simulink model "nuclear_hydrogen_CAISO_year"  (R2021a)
settings: Solver=ode23s  StartTime=0  StopTime=31618800  MaxStep=60  RelTol=2e-3
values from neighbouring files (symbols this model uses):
  alpha_f = -1.98e-5/beta    (= -0.00282857142857)    [parameter_s5.m]
  alpha_m = -28.2e-5/beta    (= -0.0402857142857)    [parameter_s5.m]
  As = n_rod*(height*2*pi*r_pellet + 2*pi*r_pellet^2)    (= 584.56254954)    [parameter_s5.m]
  beta = 0.0070    (= 0.007)    [parameter_s5.m]    (also in XSteam.m = 0)
  Cp_H2 = readmatrix('Cp.xlsx')    [parameter_s5.m]
  Ef = 200.7*1.6022e-13    (= 3.2156154e-11)    [parameter_s5.m]
  h = Nu*kappa_m/Dh    (= 9811.48906394)    [parameter_s5.m]    (also in XSteam.m = [5219.76331549428,5206.09634477373,6583.80290533381])
  k_H2 = xlsread('Hydrogen thermal conductivities.xlsx')    [parameter_s5.m]
  Lambda = 2.18e-5    (= 2.18e-05)    [parameter_s5.m]
  lambdaC = 7.728e-2    (= 0.07728)    [parameter_s5.m]
  m = Mf*1000*4/100    (= 368875.1038)    [parameter_s5.m]
  Mf = 37*249.239935    (= 9221.877595)    [parameter_s5.m]
  Mm = rho_m*V    (= 10677.6636904)    [parameter_s5.m]
  mu_H2 = xlsread('Hydrogen density.xlsx')    [parameter_s5.m]
  MW = 235.043    [parameter_s5.m]
  NA = 6.0221409e23    (= 6.0221409e+23)    [parameter_s5.m]
  p0 = -0.0065    [parameter_s5.m]
  p1 = -0.440    (= -0.44)    [parameter_s5.m]    (also in XSteam.m = p1_hs(h, s))
  p2 = -0.966    [parameter_s5.m]    (also in XSteam.m = p2_hs(h, s))
  phi0 = 9.04e+12    (= 9040000000000)    [parameter_s5.m]
  r_clad = 0.0609e-2    (= 0.000609)    [parameter_s5.m]
  r_pellet = 0.4751e-2    (= 0.004751)    [parameter_s5.m]
  rho_H2 = xlsread('Hydrogen density.xlsx')    [parameter_s5.m]
  sigmaN = 585e-24    (= 5.85e-22)    [parameter_s5.m]
  Tf0 = 719    [parameter_s5.m]
  Tm0 = 283.37    [parameter_s5.m]
libraries: pid_lib x4

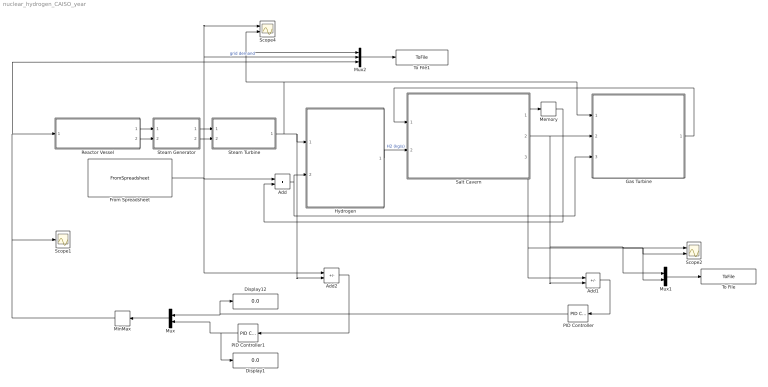
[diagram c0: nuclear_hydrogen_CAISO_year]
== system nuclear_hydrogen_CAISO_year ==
  Add : Sum
  Add1 : Sum  Inputs=+-
  Add2 : Sum  Inputs=+-
  Display1 : Display
  Display12 : Display
  From Spreadsheet : FromSpreadsheet  FileName=HistoricalEMSHourlyLoad-2020.xlsx  SheetName=data
  Gas Turbine : Subsystem
  Hydrogen : Subsystem
  Memory : Memory
  MinMax : MinMax
  Mux : Mux  Inputs=2
  Mux1 : Mux  Inputs=2
  Mux2 : Mux  Inputs=3
  PID Controller : pid_lib/PID Controller  Controller=PID  Form=Parallel  TimeDomain=Continuous-time  UseExternalTs=off  SampleTime=-1  IntegratorMethod=Forward Euler  FilterMethod=Forward Euler  ControllerParametersSource=internal  P=-1e-7  I=-5e-8  D=0  UseFilter=on  N=100  TunerSelectOption=Transfer Function Based (PID Tuner App)  InitialConditionSource=internal  InitialConditionForIntegrator=0  InitialConditionForFilter=0  DifferentiatorICPrevScaledInput=0  ExternalReset=none  TrackingMode=off  Kt=1  LimitOutput=on  SatLimitsSource=internal  UpperSaturationLimit=2  LowerSaturationLimit=0  LinearizeAsGain=on  AntiWindupMode=clamping  Kb=1  POutMin=[]  POutMax=[]  IOutMin=[]  IOutMax=[]  DOutMin=[]  DOutMax=[]  NOutMin=[]  NOutMax=[]  SumOutMin=[]  SumOutMax=[]  SaturationOutMin=[]  SaturationOutMax=[]  PParamMin=[]  PParamMax=[]  IParamMin=[]  IParamMax=[]  DParamMin=[]  DParamMax=[]  NParamMin=[]  NParamMax=[]  KbParamMin=[]  KbParamMax=[]  KtParamMin=[]  KtParamMax=[]  KbOutMin=[]  KbOutMax=[]  KtOutMin=[]  KtOutMax=[]  IntegratorOutMin=[]  IntegratorOutMax=[]  FilterOutMin=[]  FilterOutMax=[]  SumI1OutMin=[]  SumI1OutMax=[]  SumI2OutMin=[]  SumI2OutMax=[]  SumI3OutMin=[]  SumI3OutMax=[]  SumI4OutMin=[]  SumI4OutMax=[]  SumDOutMin=[]  SumDOutMax=[]  DifferentiatorOutMin=[]  DifferentiatorOutMax=[]  FilterDiffOutCoefMin=[]  FilterDiffOutCoefMax=[]  ReciprocalOutMin=[]  ReciprocalOutMax=[]  SumDenOutMin=[]  SumDenOutMax=[]  SumNumOutMin=[]  SumNumOutMax=[]  DivideOutMin=[]  DivideOutMax=[]  UdiffTsProdOutMin=[]  UdiffTsProdOutMax=[]  NTsProdOutMin=[]  NTsProdOutMax=[]  UintegralTsProdOutMin=[]  UintegralTsProdOutMax=[]  UngainTsProdOutMin=[]  UngainTsProdOutMax=[]  IntegratorContinuousStateAttributes=''  IntegratorStateMustResolveToSignalObject=off  IntegratorRTWStateStorageClass=Auto  FilterContinuousStateAttributes=''  FilterStateMustResolveToSignalObject=off  FilterRTWStateStorageClass=Auto  ParallelPVariant=InternalParameters  IdealPVariant=Disabled  IVariant=InternalParameters  DVariant=InternalParameters  IntegratorVariant=Continuous  SatVariant=Enabled  AWVariant=ContClampingParallel  PCopyVariant=Disabled  TRVariant=Disabled  FdbkBlocksVariant=Forward  IdealPFdbkVariant=Disabled  SatFdbkVariant=Disabled  DerivativeFilterVariant=ContFilter  NVariant=InternalParameters  NCopyVariant=Disabled  FilterICVariant=InternalICsFilter  IntegratorICVariant=InternalICs  ExternalResetVariant=Disabled  TRSumVariant=Passthrough  SumFdbkVariant=Disabled  SumVariant=Sum_PID  TsampFilterVariant=InternalTs  TsampNgainVariant=Passthrough  TsampIntegralVariant=Passthrough  ExternalSaturationOutDataTypeStr=Inherit: Same as second input
  PID Controller1 : pid_lib/PID Controller  Controller=PID  Form=Parallel  TimeDomain=Continuous-time  UseExternalTs=off  SampleTime=-1  IntegratorMethod=Forward Euler  FilterMethod=Forward Euler  ControllerParametersSource=internal  P=-0.067  I=-0.0044  D=0  UseFilter=on  N=100  TunerSelectOption=Transfer Function Based (PID Tuner App)  InitialConditionSource=internal  InitialConditionForIntegrator=0  InitialConditionForFilter=0  DifferentiatorICPrevScaledInput=0  ExternalReset=none  TrackingMode=off  Kt=1  LimitOutput=on  SatLimitsSource=internal  UpperSaturationLimit=2  LowerSaturationLimit=0  LinearizeAsGain=on  AntiWindupMode=clamping  Kb=1  POutMin=[]  POutMax=[]  IOutMin=[]  IOutMax=[]  DOutMin=[]  DOutMax=[]  NOutMin=[]  NOutMax=[]  SumOutMin=[]  SumOutMax=[]  SaturationOutMin=[]  SaturationOutMax=[]  PParamMin=[]  PParamMax=[]  IParamMin=[]  IParamMax=[]  DParamMin=[]  DParamMax=[]  NParamMin=[]  NParamMax=[]  KbParamMin=[]  KbParamMax=[]  KtParamMin=[]  KtParamMax=[]  KbOutMin=[]  KbOutMax=[]  KtOutMin=[]  KtOutMax=[]  IntegratorOutMin=[]  IntegratorOutMax=[]  FilterOutMin=[]  FilterOutMax=[]  SumI1OutMin=[]  SumI1OutMax=[]  SumI2OutMin=[]  SumI2OutMax=[]  SumI3OutMin=[]  SumI3OutMax=[]  SumI4OutMin=[]  SumI4OutMax=[]  SumDOutMin=[]  SumDOutMax=[]  DifferentiatorOutMin=[]  DifferentiatorOutMax=[]  FilterDiffOutCoefMin=[]  FilterDiffOutCoefMax=[]  ReciprocalOutMin=[]  ReciprocalOutMax=[]  SumDenOutMin=[]  SumDenOutMax=[]  SumNumOutMin=[]  SumNumOutMax=[]  DivideOutMin=[]  DivideOutMax=[]  UdiffTsProdOutMin=[]  UdiffTsProdOutMax=[]  NTsProdOutMin=[]  NTsProdOutMax=[]  UintegralTsProdOutMin=[]  UintegralTsProdOutMax=[]  UngainTsProdOutMin=[]  UngainTsProdOutMax=[]  IntegratorContinuousStateAttributes=''  IntegratorStateMustResolveToSignalObject=off  IntegratorRTWStateStorageClass=Auto  FilterContinuousStateAttributes=''  FilterStateMustResolveToSignalObject=off  FilterRTWStateStorageClass=Auto  ParallelPVariant=InternalParameters  IdealPVariant=Disabled  IVariant=InternalParameters  DVariant=InternalParameters  IntegratorVariant=Continuous  SatVariant=Enabled  AWVariant=ContClampingParallel  PCopyVariant=Disabled  TRVariant=Disabled  FdbkBlocksVariant=Forward  IdealPFdbkVariant=Disabled  SatFdbkVariant=Disabled  DerivativeFilterVariant=ContFilter  NVariant=InternalParameters  NCopyVariant=Disabled  FilterICVariant=InternalICsFilter  IntegratorICVariant=InternalICs  ExternalResetVariant=Disabled  TRSumVariant=Passthrough  SumFdbkVariant=Disabled  SumVariant=Sum_PID  TsampFilterVariant=InternalTs  TsampNgainVariant=Passthrough  TsampIntegralVariant=Passthrough  ExternalSaturationOutDataTypeStr=Inherit: Same as second input
  Reactor Vessel : Subsystem
  Salt Cavern : Subsystem
  Scope1 : Scope
  Scope2 : Scope  NumInputPorts=2
  Scope4 : Scope  NumInputPorts=2
  Steam Generator : Subsystem
  Steam Turbine : Subsystem
  To File : ToFile  Filename=CAISO_Cavern_Pressure_year.mat  MatrixName=ans_Pcav  SaveFormat=Timeseries
  To File1 : ToFile  Filename=CAISO_nuclear_year.mat  MatrixName=ans_NR  SaveFormat=Timeseries
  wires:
  Reactor Vessel/2(Tm) -> Steam Generator/2(Tmin)
  Reactor Vessel/1(mdot_l) -> Steam Generator/1(mdot_l)
  Hydrogen/1(Total_H2) -> Salt Cavern/2(H2_in (kg/s))  "H2 (kg/s)"
  MinMax/1 -> Scope1/1, Mux2/3, Reactor Vessel/1(control rod position (m))
  Steam Generator/1(T_steam) -> Steam Turbine/1(T1_in)
  Steam Generator/2(m_steam) -> Steam Turbine/2(m_steam)
  Add/1 -> Gas Turbine/3(grid_demand), Hydrogen/2(demand)
  Salt Cavern/1(Power_comp) -> Memory/1
  Memory/1 -> Add/2
  From Spreadsheet/1 -> Mux2/2, Scope4/1, Add2/1, Add/1  "grid demand"
  Gas Turbine/1(m_fuel) -> Salt Cavern/1(H2_out (kg/s))
  PID Controller/1 -> Display12/1, Mux/1
  PID Controller1/1 -> Display1/1, Mux/2
  Mux/1 -> MinMax/1
  Add2/1 -> PID Controller1/1
  Add1/1 -> PID Controller/1
  Salt Cavern/2(Cavern Pressure) -> Add1/2, Mux1/1, Scope2/1, Gas Turbine/2(Cavern_Pressure)
  Mux1/1 -> To File/1
  Steam Turbine/1(W_Rankine) -> Hydrogen/1(W_Rankine), Add2/2, Gas Turbine/1(Steam_Turb), Scope4/2, Mux2/1
  Mux2/1 -> To File1/1
  Salt Cavern/3(Max Pressure) -> Mux1/2, Scope2/2, Add1/1

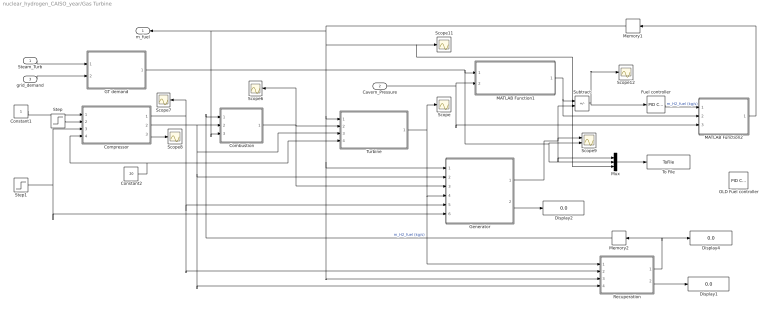
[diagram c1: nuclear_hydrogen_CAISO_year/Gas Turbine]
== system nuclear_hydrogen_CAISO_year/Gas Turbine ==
  Steam_Turb : Inport
  Cavern_Pressure : Inport  Port=2
  grid_demand : Inport  Port=3
  Combustion : MATLAB Function  TreatAsAtomicUnit=on
  Compressor : MATLAB Function  TreatAsAtomicUnit=on
  Constant1 : Constant
  Constant2 : Constant  Value=20
  Display1 : Display
  Display2 : Display
  Display4 : Display
  Fuel controller : pid_lib/PID Controller  Controller=PID  Form=Ideal  TimeDomain=Continuous-time  UseExternalTs=off  SampleTime=-1  IntegratorMethod=Forward Euler  FilterMethod=Forward Euler  ControllerParametersSource=internal  P=1e-4  I=1.2e-1  D=0  UseFilter=on  N=100  TunerSelectOption=Frequency Response Based  InitialConditionSource=internal  InitialConditionForIntegrator=0  InitialConditionForFilter=0  DifferentiatorICPrevScaledInput=0  ExternalReset=none  TrackingMode=off  Kt=1  LimitOutput=on  SatLimitsSource=internal  UpperSaturationLimit=0.2  LowerSaturationLimit=0.05236  LinearizeAsGain=on  AntiWindupMode=clamping  Kb=1  POutMin=[]  POutMax=[]  IOutMin=[]  IOutMax=[]  DOutMin=[]  DOutMax=[]  NOutMin=[]  NOutMax=[]  SumOutMin=[]  SumOutMax=[]  SaturationOutMin=[]  SaturationOutMax=[]  PParamMin=[]  PParamMax=[]  IParamMin=[]  IParamMax=[]  DParamMin=[]  DParamMax=[]  NParamMin=[]  NParamMax=[]  KbParamMin=[]  KbParamMax=[]  KtParamMin=[]  KtParamMax=[]  KbOutMin=[]  KbOutMax=[]  KtOutMin=[]  KtOutMax=[]  IntegratorOutMin=[]  IntegratorOutMax=[]  FilterOutMin=[]  FilterOutMax=[]  SumI1OutMin=[]  SumI1OutMax=[]  SumI2OutMin=[]  SumI2OutMax=[]  SumI3OutMin=[]  SumI3OutMax=[]  SumI4OutMin=[]  SumI4OutMax=[]  SumDOutMin=[]  SumDOutMax=[]  DifferentiatorOutMin=[]  DifferentiatorOutMax=[]  FilterDiffOutCoefMin=[]  FilterDiffOutCoefMax=[]  ReciprocalOutMin=[]  ReciprocalOutMax=[]  SumDenOutMin=[]  SumDenOutMax=[]  SumNumOutMin=[]  SumNumOutMax=[]  DivideOutMin=[]  DivideOutMax=[]  UdiffTsProdOutMin=[]  UdiffTsProdOutMax=[]  NTsProdOutMin=[]  NTsProdOutMax=[]  UintegralTsProdOutMin=[]  UintegralTsProdOutMax=[]  UngainTsProdOutMin=[]  UngainTsProdOutMax=[]  IntegratorContinuousStateAttributes=''  IntegratorStateMustResolveToSignalObject=off  IntegratorRTWStateStorageClass=Auto  FilterContinuousStateAttributes=''  FilterStateMustResolveToSignalObject=off  FilterRTWStateStorageClass=Auto  ParallelPVariant=Passthrough  IdealPVariant=InternalParameters  IVariant=InternalParameters  DVariant=InternalParameters  IntegratorVariant=Continuous  SatVariant=Enabled  AWVariant=ContClampingIdeal  PCopyVariant=InternalParamsIdeal  TRVariant=Disabled  FdbkBlocksVariant=Forward  IdealPFdbkVariant=Disabled  SatFdbkVariant=Disabled  DerivativeFilterVariant=ContFilter  NVariant=InternalParameters  NCopyVariant=Disabled  FilterICVariant=InternalICsFilter  IntegratorICVariant=InternalICs  ExternalResetVariant=Disabled  TRSumVariant=Passthrough  SumFdbkVariant=Disabled  SumVariant=Sum_PID  TsampFilterVariant=InternalTs  TsampNgainVariant=Passthrough  TsampIntegralVariant=Passthrough  ExternalSaturationOutDataTypeStr=Inherit: Same as second input
  GT demand : MATLAB Function  TreatAsAtomicUnit=on
  Generator : MATLAB Function  TreatAsAtomicUnit=on
  MATLAB Function1 : MATLAB Function  TreatAsAtomicUnit=on
  MATLAB Function2 : MATLAB Function  TreatAsAtomicUnit=on
  Memory1 : Memory
  Memory2 : Memory
  Mux : Mux  Inputs=3
  OLD Fuel controller : pid_lib/PID Controller  Controller=PID  Form=Ideal  TimeDomain=Continuous-time  UseExternalTs=off  SampleTime=-1  IntegratorMethod=Forward Euler  FilterMethod=Forward Euler  ControllerParametersSource=internal  P=1e-3  I=1e-2  D=0  UseFilter=on  N=100  TunerSelectOption=Frequency Response Based  InitialConditionSource=internal  InitialConditionForIntegrator=0  InitialConditionForFilter=0  DifferentiatorICPrevScaledInput=0  ExternalReset=none  TrackingMode=off  Kt=1  LimitOutput=on  SatLimitsSource=internal  UpperSaturationLimit=0.2  LowerSaturationLimit=0.05236  LinearizeAsGain=on  AntiWindupMode=clamping  Kb=1  POutMin=[]  POutMax=[]  IOutMin=[]  IOutMax=[]  DOutMin=[]  DOutMax=[]  NOutMin=[]  NOutMax=[]  SumOutMin=[]  SumOutMax=[]  SaturationOutMin=[]  SaturationOutMax=[]  PParamMin=[]  PParamMax=[]  IParamMin=[]  IParamMax=[]  DParamMin=[]  DParamMax=[]  NParamMin=[]  NParamMax=[]  KbParamMin=[]  KbParamMax=[]  KtParamMin=[]  KtParamMax=[]  KbOutMin=[]  KbOutMax=[]  KtOutMin=[]  KtOutMax=[]  IntegratorOutMin=[]  IntegratorOutMax=[]  FilterOutMin=[]  FilterOutMax=[]  SumI1OutMin=[]  SumI1OutMax=[]  SumI2OutMin=[]  SumI2OutMax=[]  SumI3OutMin=[]  SumI3OutMax=[]  SumI4OutMin=[]  SumI4OutMax=[]  SumDOutMin=[]  SumDOutMax=[]  DifferentiatorOutMin=[]  DifferentiatorOutMax=[]  FilterDiffOutCoefMin=[]  FilterDiffOutCoefMax=[]  ReciprocalOutMin=[]  ReciprocalOutMax=[]  SumDenOutMin=[]  SumDenOutMax=[]  SumNumOutMin=[]  SumNumOutMax=[]  DivideOutMin=[]  DivideOutMax=[]  UdiffTsProdOutMin=[]  UdiffTsProdOutMax=[]  NTsProdOutMin=[]  NTsProdOutMax=[]  UintegralTsProdOutMin=[]  UintegralTsProdOutMax=[]  UngainTsProdOutMin=[]  UngainTsProdOutMax=[]  IntegratorContinuousStateAttributes=''  IntegratorStateMustResolveToSignalObject=off  IntegratorRTWStateStorageClass=Auto  FilterContinuousStateAttributes=''  FilterStateMustResolveToSignalObject=off  FilterRTWStateStorageClass=Auto  ParallelPVariant=Passthrough  IdealPVariant=InternalParameters  IVariant=InternalParameters  DVariant=InternalParameters  IntegratorVariant=Continuous  SatVariant=Enabled  AWVariant=ContClampingIdeal  PCopyVariant=InternalParamsIdeal  TRVariant=Disabled  FdbkBlocksVariant=Forward  IdealPFdbkVariant=Disabled  SatFdbkVariant=Disabled  DerivativeFilterVariant=ContFilter  NVariant=InternalParameters  NCopyVariant=Disabled  FilterICVariant=InternalICsFilter  IntegratorICVariant=InternalICs  ExternalResetVariant=Disabled  TRSumVariant=Passthrough  SumFdbkVariant=Disabled  SumVariant=Sum_PID  TsampFilterVariant=InternalTs  TsampNgainVariant=Passthrough  TsampIntegralVariant=Passthrough  ExternalSaturationOutDataTypeStr=Inherit: Same as second input
  Recuperation : MATLAB Function  TreatAsAtomicUnit=on
  Scope{,6..8,11..12} (6 alike) : Scope
  Scope9 : Scope  NumInputPorts=2
  Step : Step  Time=4  Before=80  After=80  SampleTime=0
  Step1 : Step  Time=7  Before=280  After=280  SampleTime=0
  Subtract : Sum  Inputs=+-
  To File : ToFile  Filename=CAISO_GT_Power_year.mat  MatrixName=ans_GT  SaveFormat=Timeseries
  Turbine : MATLAB Function  TreatAsAtomicUnit=on
  m_fuel : Outport
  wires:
  Combustion/1(T_f) -> Generator/3(T_f), Scope6/1, Turbine/2(T_f)
  Constant2/1 -> Compressor/4(m_an), Turbine/4(m_an)
  GT demand/1(GT_demand) -> Mux/2, Scope9/2, MATLAB Function1/1(SP)
  Fuel controller/1 -> MATLAB Function2/1(m_f)  "m_H2_fuel (kg/s)"
  MATLAB Function1/1(Set_point) -> MATLAB Function2/2(GT_SP), Subtract/1
  Generator/1(P_overall) -> Mux/1, Scope9/1, Subtract/2
  Steam_Turb/1 -> GT demand/1(Steam_Turb)
  Cavern_Pressure/1 -> MATLAB Function2/3(Cavern_P), MATLAB Function1/2(Cavern_Pressure)
  Step1/1 -> Generator/6(T_amb), Compressor/3(T_amb)
  Constant1/1 -> Compressor/1(P_amb)
  Subtract/1 -> Scope12/1, Fuel controller/1
  Step/1 -> Compressor/2(theta_IGV)
  Compressor/3(P_out) -> Scope8/1
  grid_demand/1 -> GT demand/2(grid_demand)
  Compressor/1(Td) -> Recuperation/2(T_d), Generator/5(T_d), Scope7/1
  Turbine/1(T_e) -> Scope/1, Recuperation/1(T_e), Generator/4(T_e)
  Recuperation/1(Tc_in) -> Display4/1, Memory2/1
  Compressor/2(m_a) -> Recuperation/4(m_a), Generator/2(m_a), Turbine/3(m_a), Combustion/2(m_a)
  Memory2/1 -> Combustion/1(T_d)  "m_H2_fuel (kg/s)"
  Recuperation/2(T_6) -> Display1/1
  Generator/2(efficiency) -> Display2/1
  Mux/1 -> To File/1
  Memory1/1 -> Combustion/3(m_f), m_fuel/1, Mux/3, Scope11/1, Recuperation/3(m_f), Generator/1(m_f), Turbine/1(m_f)
  MATLAB Function2/1(m_H2) -> Memory1/1

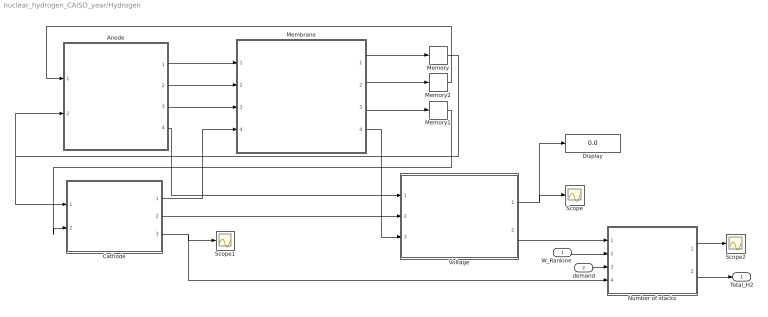
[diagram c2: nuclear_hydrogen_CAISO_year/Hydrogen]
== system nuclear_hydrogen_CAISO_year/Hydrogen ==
  W_Rankine : Inport
  demand : Inport  Port=2
  Anode : MATLAB Function  TreatAsAtomicUnit=on
  Cathode : MATLAB Function  TreatAsAtomicUnit=on
  Display : Display
  Membrane : MATLAB Function  TreatAsAtomicUnit=on
  Memory : Memory
  Memory1 : Memory
  Memory2 : Memory
  Number of stacks : MATLAB Function  TreatAsAtomicUnit=on
  Scope : Scope
  Scope1 : Scope
  Scope2 : Scope
  Voltage : MATLAB Function  TreatAsAtomicUnit=on
  Total_H2 : Outport
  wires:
  Memory/1 -> Anode/2(F_H2O_m), Cathode/1(F_H2O_m)
  Cathode/1(nH2O_cat) -> Membrane/4(n_H2O_c)
  Anode/1(nH2O_an) -> Membrane/1(n_H2O_a)
  Membrane/1(FH2Om) -> Memory/1
  Cathode/2(P_H2) -> Voltage/2(P_H2)
  Cathode/3(dNH2dt) -> Number of stacks/4(n_H2), Scope1/1
  Memory1/1 -> Cathode/2(D_cat)
  Memory2/1 -> Anode/1(D_an)
  Anode/4(P_O2) -> Voltage/1(P_O2)
  Voltage/1(V) -> Display/1, Scope/1
  Membrane/3(D_cat) -> Memory1/1
  Membrane/2(D_an) -> Memory2/1
  Membrane/4(PH2O_me_an) -> Voltage/3(P_H2O)
  Anode/2(F_H2O_cons) -> Membrane/2(FH2O_cons)
  Anode/3(CO2_me) -> Membrane/3(CO2_me)
  Voltage/2(Power) -> Number of stacks/1(Power)
  W_Rankine/1 -> Number of stacks/2(P_Turb)
  Number of stacks/2(Total_H2) -> Total_H2/1
  demand/1 -> Number of stacks/3(demand)
  Number of stacks/1(n) -> Scope2/1

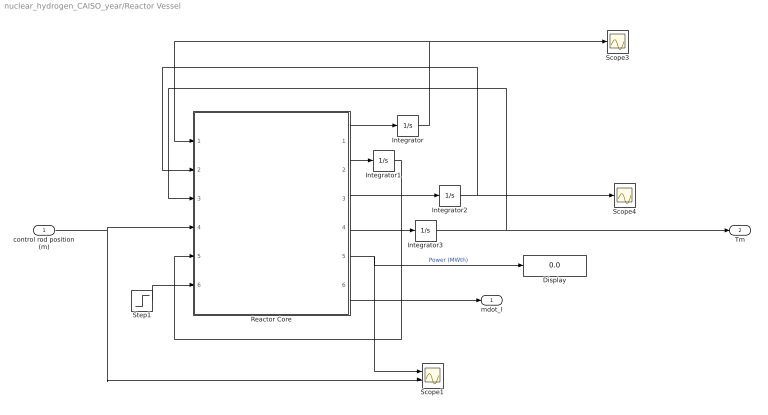
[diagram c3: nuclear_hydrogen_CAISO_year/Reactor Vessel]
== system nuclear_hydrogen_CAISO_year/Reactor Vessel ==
  control rod position (m) : Inport
  Display : Display
  Integrator : Integrator  InitialCondition=99.35
  Integrator1 : Integrator  InitialCondition=.65
  Integrator2 : Integrator  InitialCondition=719
  Integrator3 : Integrator  InitialCondition=284
  Reactor Core : MATLAB Function  TreatAsAtomicUnit=on
  Scope1 : Scope  NumInputPorts=2
  Scope3 : Scope
  Scope4 : Scope
  Step1 : Step  Time=6  Before=258.3  After=258.3  SampleTime=0
  mdot_l : Outport
  Tm : Outport  Port=2
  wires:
  Integrator1/1 -> Reactor Core/5(C)
  Integrator2/1 -> Scope4/1, Reactor Core/2(Tf)
  Integrator/1 -> Reactor Core/1(N), Scope3/1
  Reactor Core/2(dCdt) -> Integrator1/1
  Reactor Core/1(dNdt) -> Integrator/1
  Reactor Core/5(Power) -> Scope1/1, Display/1  "Power (MWth)"
  control rod position (m)/1 -> Scope1/2, Reactor Core/4(z)
  Reactor Core/3(dTfdt) -> Integrator2/1
  Integrator3/1 -> Tm/1, Reactor Core/3(Tm)
  Reactor Core/4(dTmdt) -> Integrator3/1
  Step1/1 -> Reactor Core/6(Tin)
  Reactor Core/6(mdot_l) -> mdot_l/1

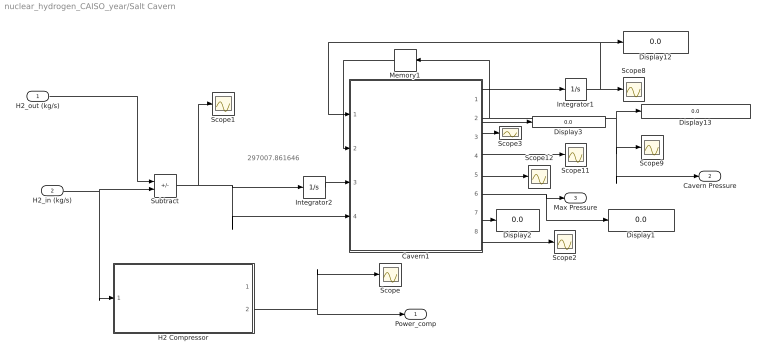
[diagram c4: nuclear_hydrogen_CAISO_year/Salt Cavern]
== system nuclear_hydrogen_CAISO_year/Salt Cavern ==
  note: 297007.861646
  H2_out (kg/s) : Inport
  H2_in (kg/s) : Inport  Port=2
  Cavern1 : MATLAB Function  TreatAsAtomicUnit=on
  Display{1..3,12..13} (5 alike) : Display
  H2 Compressor : MATLAB Function  TreatAsAtomicUnit=on
  Integrator1 : Integrator  InitialCondition=313.15
  Integrator2 : Integrator  InitialCondition=297007.861646
  Memory1 : Memory
  Scope{,1..3,8..9,11..12} (8 alike) : Scope
  Subtract : Sum  Inputs=-+
  Power_comp : Outport
  Cavern Pressure : Outport  Port=2
  Max Pressure : Outport  Port=3
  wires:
  Cavern1/4(z) -> Scope11/1
  Cavern1/2(P) -> Cavern Pressure/1, Scope9/1, Display13/1, Memory1/1
  H2_in (kg/s)/1 -> H2 Compressor/1(nH2), Subtract/2
  Cavern1/1(dTdt) -> Integrator1/1
  Integrator1/1 -> Scope8/1, Display12/1, Cavern1/1(T)
  Memory1/1 -> Cavern1/2("P ")
  Integrator2/1 -> Cavern1/3(m)
  Cavern1/5(lambda) -> Scope12/1
  H2 Compressor/2(Total_P) -> Scope/1, Power_comp/1
  H2_out (kg/s)/1 -> Subtract/1
  Subtract/1 -> Scope1/1, Integrator2/1, Cavern1/4(mH2_in)
  Cavern1/6(P_max) -> Display1/1, Max Pressure/1
  Cavern1/7(P_min) -> Display2/1
  Cavern1/8(Cp) -> Scope2/1
  Cavern1/3(n) -> Display3/1, Scope3/1

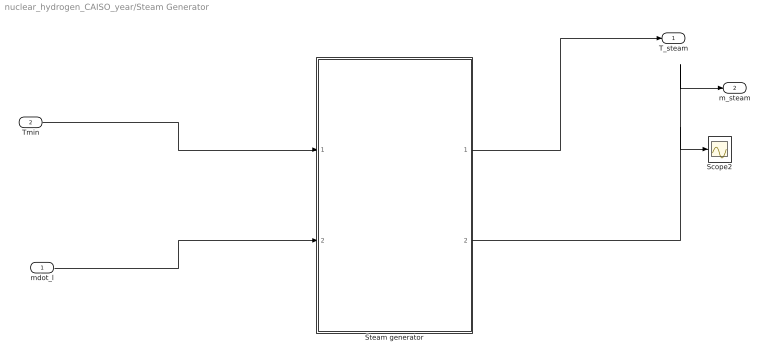
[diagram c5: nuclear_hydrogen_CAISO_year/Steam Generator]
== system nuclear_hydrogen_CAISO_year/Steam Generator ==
  mdot_l : Inport
  Tmin : Inport  Port=2
  Scope2 : Scope
  Steam generator : MATLAB Function  TreatAsAtomicUnit=on
  T_steam : Outport
  m_steam : Outport  Port=2
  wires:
  Steam generator/2(m_steam) -> m_steam/1, Scope2/1
  Tmin/1 -> Steam generator/1(Tmin)
  mdot_l/1 -> Steam generator/2(mdot_l)
  Steam generator/1(T_steam_out) -> T_steam/1

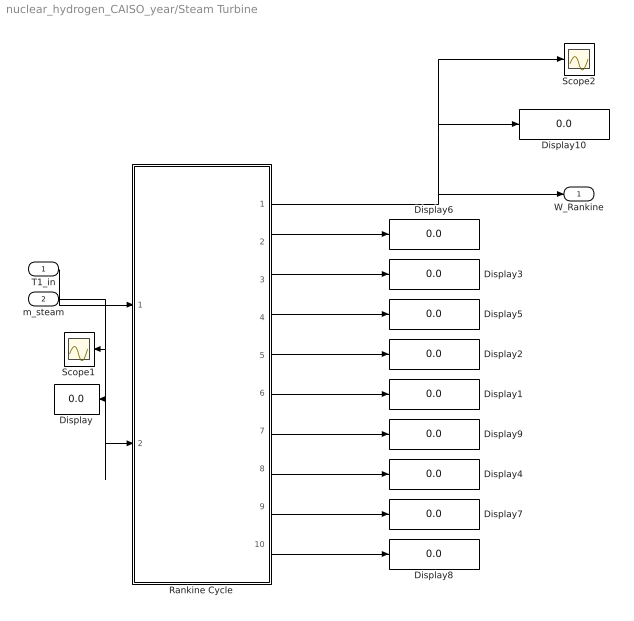
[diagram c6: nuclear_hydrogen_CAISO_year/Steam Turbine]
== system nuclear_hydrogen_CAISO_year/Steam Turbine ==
  T1_in : Inport
  m_steam : Inport  Port=2
  Display{,1..10} (11 alike) : Display
  Rankine Cycle : MATLAB Function  TreatAsAtomicUnit=on
  Scope1 : Scope
  Scope2 : Scope
  W_Rankine : Outport
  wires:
  Rankine Cycle/2(W_T1) -> Display6/1
  Rankine Cycle/9(W_p1) -> Display7/1
  Rankine Cycle/8(T_p1_out) -> Display4/1
  Rankine Cycle/5(T1_out) -> Display2/1
  Rankine Cycle/10(T_fwh1_out) -> Display8/1
  Rankine Cycle/4(h1_out) -> Display5/1
  Rankine Cycle/6(Tsat_1) -> Display1/1
  Rankine Cycle/3(P1_out) -> Display3/1
  Rankine Cycle/7(q_cond) -> Display9/1
  m_steam/1 -> Rankine Cycle/2(m_steam), Display/1, Scope1/1
  T1_in/1 -> Rankine Cycle/1(T1_in)
  Rankine Cycle/1(Power) -> Display10/1, Scope2/1, W_Rankine/1

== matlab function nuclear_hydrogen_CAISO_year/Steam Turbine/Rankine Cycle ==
function [Power, W_T1,P1_out,h1_out,T1_out,Tsat_1,q_cond,T_p1_out,W_p1,T_fwh1_out] = T1_ex(T1_in,m_steam)
coder.extrinsic('XSteam.m');
eta_turb = 0.75;
eta_pump = 0.70;
TTD = 0.1;
P1_in = 34.6; % bar turbine inlet pressure https://inldigitallibrary.inl.gov/sites/sti/sti/Sort_20117.pdf
Tsat_hi = XSteam('Tsat_p', P1_in);
Tsat_lo = XSteam('Tsat_p', 0.25);
%% Turbine inlet conditions
h_in            = XSteam('h_pT',P1_in,T1_in);       % inlet enthalpy (kJ/kg)
s_in            = XSteam('s_pT',P1_in,T1_in);       % inlet entropy (kJ/kg°C)
%% HP turbine outlet conditions
P1_out         = 0.066;                                           % outlet pressure (bar) https://www.nuclear-power.net/nuclear-engineering/thermodynamics/thermodynamic-cycles/rankine-cycle-steam-turbine-cycle/boiler-and-condenser-pressures-rankine-cycle/#:~:text=The%20lowest%20feasible%20condenser%20pressure,in%20a%20thermal%20power%20plant.
h_out_id       = XSteam('h_ps',P1_out,s_in);                     % ideal outlet enthalpy (kJ/kg)
h1_out         = h_in + eta_turb*(h_out_id - h_in);              % actual outlet enthalpy (kJ/kg)
T1_out         = XSteam('T_ph',P1_out,h1_out);                   % outlet T based on enthalpy (kJ/kg)
s1_out         = XSteam('s_ph',P1_out,h1_out);
Tsat_1         = XSteam('Tsat_p',P1_out);
W_T1           = m_steam*(h_in - h1_out)/1e3;                    % Work rate (MW)
%% Condenser
Pc_out          = P1_out;                                % outlet pressure of condensor (bar)
Tc_out          = XSteam('Tsat_p',Pc_out) - 0.5;         % outlet temperature condensor, slightly subcooled from saturation
hc_out          = XSteam('h_pT',Pc_out,Tc_out);          % outlet enthalpy (kJ/kg)
sc_out          = XSteam('s_pT',Pc_out,Tc_out);          % outlet entropy (kJ/kg°C)
vc_out          = XSteam('v_pT',Pc_out,Tc_out);          % specific volume outlet (m^3/kg)
q_cond          = m_steam*(h1_out - hc_out)/1e3;         % heat rejection rate (MJ/kg)
%% Pump1
P_p1_out        = P1_in;                                 % outlet Pressure (bar), same as outlet of turbine 2
v_p1            = vc_out;                                % inlet specific volume (m^3/kg)
W_p1            = m_steam*v_p1*(Pc_out - P_p1_out)*1e5/eta_pump/1e6;
%Parastic work of pump 1 (MW)
h_p1_out        = hc_out - W_p1*1e3/m_steam;             % outlet enthalpy (kJ/kg)
T_p1_out        = XSteam('T_ph',P_p1_out,h_p1_out);      % outlet temperature (C)
%% FWH 1
T_fwh1_out      = XSteam('Tsat_p',P_p1_out) - TTD;         % outlet temperature based upon TTD method (K)
h_fwh1_out      = XSteam('h_pT',P_p1_out,T_fwh1_out);      % outlet enthalpy of preheater (kJ/kg)
v_fwh1_out      = XSteam('v_ph', P_p1_out, h_fwh1_out);    % specific volume outlet (m^3/kg)
z_est           = (h_fwh1_out - h_p1_out)/(h1_out - h_p1_out);
z_est(isnan(z_est)) = 0.05;
z_est(z_est>1)  = 0.99;
z_est(z_est<0)  = 0.01;
vap_f1       	= XSteam('x_ph',Pc_out, h_fwh1_out);
%% Total power output
Power = W_T1 + W_p1;

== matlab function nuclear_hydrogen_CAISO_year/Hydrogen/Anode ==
function [nH2O_an, F_H2O_cons, CO2_me, P_O2] = fcn(D_an, F_H2O_m)
%% Parameters
Temp    = 25; %C
Current = 80; % A
P_an    = 101325; % Pa
F          = 96485.3329; % (sA/mol) Faraday Constant
A          = 160e-4; % m2
T_an       = Temp + 273.15; % Converting from C to K
R          = 8.3145; % J/molK
d_an       = 8e-5; % anode thickness
%% O2 mass balance
FO2_in     = 0; % O2 in
FO2_gen    = Current/(4*F); % O2 generated (mol/s)
dNO2dt     = FO2_in + FO2_gen;
nO2        = dNO2dt/A; % O2 flow per unit area
%% H2O mass balance
F_H2O_cons = Current/(2*F); % water consumed (mol/s)
FH2O_an    = F_H2O_cons + F_H2O_m;
nH2O_an    = FH2O_an/A; % H2O flow per unit area in anode
%% Concentration
yO2_ch     = nO2/(nO2+nH2O_an);
yH2O_an    = nH2O_an/(nO2+nH2O_an);
CO2_ch     = P_an*yO2_ch/(R*T_an);
CO2_me     = CO2_ch + d_an*nO2/D_an;
yO2_me     = R*T_an*CO2_me/P_an;
%% Pressure
P_O2       = yO2_me*P_an;

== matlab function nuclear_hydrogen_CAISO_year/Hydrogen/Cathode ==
function [nH2O_cat, P_H2, dNH2dt] = fcn(F_H2O_m, D_cat)
%% Parameters
Temp    = 25; %C
Current = 80; % A
P_cat   = 101325; % Pa
F          = 96485.3329; % (sA/mol) Faraday Constant
A          = 160e-4; % m2
T_cat      = Temp + 273.15; % Converting from C to K
R          = 8.3145; % J/molK
d_cat      = 8e-5; % cathode thickness
%% H2 mass balance
FH2_in     = 0; % O2 in
FH2_gen    = Current/(2*F); % H2 generated (mol/s)
dNH2dt     = FH2_in + FH2_gen;
nH2        = dNH2dt/A; % H2 flow per unit area
%% H2O mass balance
FH2O_cat   = F_H2O_m;
nH2O_cat   = FH2O_cat/A; % H2O flow per unit area in cathode
%% Concentration
yH2_ch     = nH2/(nH2+nH2O_cat);
yH2O_cat   = nH2O_cat/(nH2+nH2O_cat);
CH2_ch     = P_cat*yH2_ch/(R*T_cat);
CH2_me     = CH2_ch + d_cat*nH2/D_cat;
yH2_me     = R*T_cat/P_cat*CH2_me;
%% Pressure
P_H2       = yH2_me*P_cat;

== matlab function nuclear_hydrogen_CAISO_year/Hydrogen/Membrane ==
function [FH2Om, D_an, D_cat, PH2O_me_an] = fcn(n_H2O_a, FH2O_cons, CO2_me, n_H2O_c)
%% Parameters
Temp    = 25; %C
Temp_a  = Temp;
Temp_c  = Temp;
Current = 80; % A
P_an    = 101325; % Pa
P_cat   = 101325; % Pa
F            = 96485.3329; % (sA/mol) Faraday Constant
t_me         = 0.175e-6; % m (Tevfik) membrane thickness
MWw          = 18.02e-3; % kg/mol
Tc           = Temp_c + 273.15; % Coverting cathode Temperature from C to K
Ta           = Temp_a + 273.15; % Convering anode Temperature from C to K
T            = (Tc + Ta)/2;
d_cat        = 8e-5; % cathode thickness
d_an         = 8e-5; % anode thickness
A            = 160e-4; % m2
Dw           = 1.28e-10; % m2/s Theoretical model and experimental analysis of a highpressure PEM water electrolyser for hydrogen production
K_darcy      = 1.58e-18; % m2 Theoretical model and experimental analysis of a highpressure PEM water electrolyser for hydrogen production
mu_w         = 1.1e-3; % kg/(m*s) or Pa*s
rho_w        = 1e3; % kg/m3
epsilon      = 0.3; % Theoretical model and experimental analysis of a highpressure PEM water electrolyser for hydrogen production
epsilon_p    = 0.11; % Theoretical model and experimental analysis of a highpressure PEM water electrolyser for hydrogen production
alpha        = 0.785; % Theoretical model and experimental analysis of a highpressure PEM water electrolyser for hydrogen production
a            = 3.640e-4;
b            = 2.334;
Tc_O2        = 154.4; % K
Tc_H2        = 33.3; % K
Tc_H2O       = 647.3; % K
Pc_O2        = 49.7; % atm
Pc_H2        = 12.8; % atm
Pc_H2O       = 218.3; % atm
Mm_O2        = 16; % g/mol
Mm_H2        = 2; % g/mol
Mm_H2O       = 18; % g/mol
%% Water diffusion
rho_w_c      = 0.14395/0.0112^(1+(1-Tc/649.727)^0.05107);  % kg/m3 water density in the cathode
rho_w_a      = 0.14395/0.0112^(1+(1-Ta/649.727)^0.05107);  % kg/m3 water density in the anode
Cwc_ch       = rho_w_c/MWw;
Cwa_ch       = rho_w_a/MWw;
D_AB_cat     = a*(T/sqrt(Tc_O2*Tc_H2O))^b*(Pc_O2*Pc_H2O)^(1/3)*(Tc_O2*Tc_H2O)^(5/12)*(1/Mm_O2+1/Mm_H2O)^0.5; % O2/H2O
D_AB_an      = a*(T/sqrt(Tc_H2*Tc_H2O))^b*(Pc_H2*Pc_H2O)^(1/3)*(Tc_H2*Tc_H2O)^(5/12)*(1/Mm_H2+1/Mm_H2O)^0.5; % H2/H2O
D_cat        = D_AB_cat*epsilon*((epsilon - epsilon_p)/(1-epsilon_p))^alpha;
D_an         = D_AB_an*epsilon*((epsilon - epsilon_p)/(1-epsilon_p))^alpha;
Cwc          = Cwc_ch + d_cat*n_H2O_c/D_cat; % Concentration of water at the membrane in the cathode side (CH2O_me_cat)
Cwa          = Cwa_ch - d_an*n_H2O_a/D_an; % Concentration of water at the membrane in the anode side (CH2O_me_an)
dNH2Odt_diff = A*Dw*(Cwc - Cwa)/t_me; %D_lambda     = 1.25e-10; % m2/s Dw           = D_lambda*exp(2416*(1/303-1/T));
%% Electro Osmotic Drag
nd           = 7; % Theoretical model and experimental analysis of a highpressure PEM water electrolyser for hydrogen production
dNH2Odt_eod  = nd*Current/F;
%% Hydraulic Pressure
dNH2Odt_p    = K_darcy*A*rho_w/(mu_w*MWw); % K_darcy*A*rho_w*(P_cat - P_an)/(t_me*mu_w*MWw)
%% Membrane water transport
FH2Om_A      = dNH2Odt_eod - dNH2Odt_p + A*Dw/t_me*((rho_w_c-rho_w_a)/MWw + d_an*FH2O_cons/(D_an*A));
FH2Om_B      = 1 - Dw/t_me*(d_cat/D_cat + d_an/D_an);
FH2Om        = FH2Om_A/FH2Om_B;
%% Concentration and Pressure
yH2O_me_an   = Cwa/(Cwa + CO2_me);
PH2O_me_an   = yH2O_me_an*P_an;

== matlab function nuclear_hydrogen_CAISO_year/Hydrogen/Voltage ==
function [V,Power] = fcn(P_O2,P_H2,P_H2O)
%% Parameters from Mathematical modeling and dynamic Simulink simulation of high-pressure PEM electrolyzer system
alpha_an   = 2;
alpha_cat  = 0.5;
i_knot_an  = 2e-7;
i_knot_cat = 2e-3;
Area       = 160e-4; % m2
Temp    = 25; %C
Current = 80; % A
R     = 8.3145; % m^3 Pa/mol K
T     = Temp + 273.15;
n     = 2;
F     = 96485.3329;% (s*A/mol)
%% Open-circuit voltage
E_rev = 1.229 - 0.9e-3*(Temp - 25);
E     = E_rev + R*T/(n*F)*log(P_H2*P_O2^0.5/(P_H2O)); % A review on PEM
%% Activation overvoltage
Current_Density = Current/Area;
V_act_an   = R*T/(alpha_an*F)*asinh(Current_Density/(2*i_knot_an));
V_act_cat  = R*T/(alpha_cat*F)*asinh(Current_Density/(2*i_knot_cat));
V_act      = V_act_an + V_act_cat;
%% Ohmic overvoltage
lambda   = 25;
t_me     = 0.175e-6; % m (Tevfik) membrane thickness
sigma_m  = (0.005139*lambda - 0.00326)*exp(1268*(1/303-1/T));
R_ohm    = t_me/sigma_m; 
V_ohm    = Current_Density*R_ohm;
%% Total Voltage
V          = E + V_act + V_ohm;
Power      = V*Current;

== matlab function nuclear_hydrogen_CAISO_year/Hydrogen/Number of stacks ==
function [n, Total_H2]  = fcn(Power, P_Turb, demand, n_H2)
MW_H2      = 2e-3; % kg/mol
n          = floor((P_Turb-demand)*1e6/Power);
if n<0
    n =0;
end
Total_H2   = n*n_H2*MW_H2; % kg/s;

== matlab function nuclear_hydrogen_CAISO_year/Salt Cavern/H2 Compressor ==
function [T_out, Total_P] = fcn(nH2)
MWH2     = 2;          % kg/kmol
%% Power needed to raise H2 from 1 atm to 2 MPa
Power_1  = nH2*1.02*3600*1e-3; % MW https://www.hydrogen.energy.gov/pdfs/9013_energy_requirements_for_hydrogen_gas_compression.pdf
%% Power needed to raise H2 from 2 MPa/300 K to 3.42 MPa/362 K
Power_2  = nH2*180.84*1e-3/0.2; % MW https://www.sciencedirect.com/science/article/pii/S036054421730899X#bib13
%% Power needed to raise H2 from 3.42 MPa/300 K to 5.85 MPa/363.85 K
Power_3  = nH2*187.73*1e-3/0.2; % MW https://www.sciencedirect.com/science/article/pii/S036054421730899X#bib13
%% POwer needed to raise H2 from 5.85 MPa/300 K to 10 MPa/365.65 K
Power_4  = nH2*196.1*1e-3/0.2; % MW https://www.sciencedirect.com/science/article/pii/S036054421730899X#bib13
%% Power needed to raise H2 from 10 MPa/ 300 K to 17 MPa/349.33 K
H_in     = 8.0741e+06;         % J/kmol
S_in     = 6.9427e+04;         % J/kmol/K
H_out    = 9.6114e+06;         % J/kmol same S as S_in
eta_comp = 0.56;               % compressor efficiency https://www.hydrogen.energy.gov/pdfs/9013_energy_requirements_for_hydrogen_gas_compression.pdf
nH2      = nH2/MWH2;           % converting kg/s to kmol/s
Ideal_P  = nH2*(H_out - H_in)*1e-6; % MW
Power_5  = Ideal_P/eta_comp;   % MW
%% Total Power
Total_P  = Power_1 + Power_2 + Power_3 + Power_4 + Power_5; 
T_out    = 349.33; % K

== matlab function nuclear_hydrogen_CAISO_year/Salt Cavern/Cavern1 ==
function [dTdt, P, n, z, lambda, P_max, P_min, Cp] = Cavern1(T, P, m, mH2_in,Cp_H2, rho_H2, k_H2, mu_H2)
%% Parameters
Tw       = 40 + 273.15; % K rock temperature
T0       = 313.15; % K cavern intial temperature Comprehensive modeling and developing a software for salt cavern underground gas storage
P0       = 10e6; % Pa cavern initial pressure of the cavern
R        = 8.3145; % m3*Pa/(mol*K)
H_top    = 1000; % m top depth of cavern
H_bot    = 1200; % m bottom depth of cavern
R_cavern = 16/2;   % m cavern radius
L        = H_bot - H_top;
V_cavern = L*pi*R_cavern^2; % m3
g        = 9.81; % m/s2
MW_H2    = 2e-3; % kg/mol
%% functions
z0       = comp(T0,P0);
z        = 1.04; % comp(T,P); Seasonal energy storage for...
% n0       = P0*V_cavern/(z0*R*T0);               % (mols)
Cp       = CalculateCp(T,P,Cp_H2);              % J/mol*K
% rho      = density(T,P,rho_H2)*MW_H2;           % (kg/m3)
% rho_w    = density(Tw,P,rho_H2)*MW_H2;          % (kg/m3)
% k        = thermalcond(T,P,k_H2);               % (W/m*K)
% mu       = dyn_vis(T,P,mu_H2)*1e6;              % (Pa*s)
% Ra       = g*rho*Cp*abs(rho-rho_w)*L^3/(k*mu);
% if Ra<=10e9
%     h    = k/L*(0.68 + 0.67*Ra^0.25/(1 + (0.492*k/(mu*Cp))^(9/16))^(4/9)); % W/m2*K
% else
%     h    = k/L*(0.825 + 0.387*Ra^(1/6)/(1 + (0.492*k/(mu*Cp))^(9/16))^(8/27)); % W/m2*K
% end
% Area     = L*2*pi*R_cavern;
lambda   = 8.6; %h*Area;
%% Solve for T and P
n_dot    = mH2_in/MW_H2;              % converting from kg/s to mol/s
n        = m/MW_H2;                   % converting from kg to mols
dndt     = n_dot;                     % mol/s
if n_dot >0
    H_in     = 9.8168e+03;                % J/mol at 362 K and 3.42 MPa
else
    H_in     = Cp*T;
end
dTdt     = ((n_dot*H_in + lambda*(Tw-T))/Cp-T*dndt)/n;
P        = z*n*R*T/V_cavern;          % Pa
%% Calculate P max and min
rho_rock       = 2200; % kg/m3
P_geostatic    = rho_rock*g*H_top; % Pa Technical Potential of Salt Caverns for Hydrogen Storage in Europe page 8
P_max          = 0.80*P_geostatic; % Pa
P_min          = 0.30*P_geostatic; % Pa
end
function z = comp(T,P)
a        = [0.05888460, -0.06136111, -0.002650473, 0.002731125, 0.001802374, -0.0012150707, 0.958852E-4, -0.1109040E-6, 0.1264403E-9];
b        = [1.325, 1.87, 2.5, 2.8, 2.38, 3.14, 3.37, 3.75, 4.0];
c        = [1, 1, 2, 2, 2.42, 2.63, 3, 4, 5];
z        = 1 + a(1)*(100/T)^b(1)*(P/1e6)^c(1) + ...
    a(2)*(100/T)^b(2)*(P/1e6)^c(2) + ...
    a(3)*(100/T)^b(3)*(P/1e6)^c(3) + ...
    a(4)*(100/T)^b(4)*(P/1e6)^c(4) + ...
    a(5)*(100/T)^b(5)*(P/1e6)^c(5) + ...
    a(6)*(100/T)^b(6)*(P/1e6)^c(6) + ...
    a(7)*(100/T)^b(7)*(P/1e6)^c(7) + ...
    a(8)*(100/T)^b(8)*(P/1e6)^c(8) + ...
    a(9)*(100/T)^b(9)*(P/1e6)^c(9); % compressibilty factor
end
function Out = CalculateCp(T,P,Cp)
if P<2e6
    P = 2e6;
end
Cp_Tf1 = Cp(floor(T-289),floor(P/1e6-1));
Cp_Tf2 = Cp(ceil(T-289), floor(P/1e6-1));
Cp_Tf  = (Cp_Tf2 - Cp_Tf1)*(T-floor(T)) + Cp_Tf1;

Cp_Tc1 = Cp(floor(T-289),ceil(P/1e6-1));
Cp_Tc2 = Cp(ceil(T-289), ceil(P/1e6-1));
Cp_Tc  = (Cp_Tc2 - Cp_Tc1)*(T-floor(T)) + Cp_Tc1;

Out = (Cp_Tc-Cp_Tf)*(P/1e6-floor(P/1e6)) + Cp_Tf;
end
function out = thermalcond(T,P,k)
if P<2e6
    P = 2e6;
end
k_Tf1 = k(floor(T-289),floor(P/1e6-1));
k_Tf2 = k(ceil(T-289), floor(P/1e6-1));
k_Tf  = (k_Tf2 - k_Tf1)*(T-floor(T)) + k_Tf1;

k_Tc1 = k(floor(T-289),ceil(P/1e6-1));
k_Tc2 = k(ceil(T-289), ceil(P/1e6-1));
k_Tc  = (k_Tc2 - k_Tc1)*(T-floor(T)) + k_Tc1;

out = (k_Tc-k_Tf)*(P/1e6-floor(P/1e6)) + k_Tf; % (W/m*K)
end
function out = density(T,P,rho)
if P<2e6
    P = 2e6;
end
rho_Tf1 = rho(floor(T-289),floor(P/1e6-1));
rho_Tf2 = rho(ceil(T-289), floor(P/1e6-1));
rho_Tf  = (rho_Tf2 - rho_Tf1)*(T-floor(T)) + rho_Tf1;

rho_Tc1 = rho(floor(T-289),ceil(P/1e6-1));
rho_Tc2 = rho(ceil(T-289), ceil(P/1e6-1));
rho_Tc  = (rho_Tc2 - rho_Tc1)*(T-floor(T)) + rho_Tc1;

out = (rho_Tc-rho_Tf)*(P/1e6-floor(P/1e6)) + rho_Tf; % (mol/m3)
end
function out = dyn_vis(T,P,mu)
if P<2e6
    P = 2e6;
end
mu_Tf1 = mu(floor(T-289),floor(P/1e6-1));
mu_Tf2 = mu(ceil(T-289), floor(P/1e6-1));
mu_Tf  = (mu_Tf2 - mu_Tf1)*(T-floor(T)) + mu_Tf1;

mu_Tc1 = mu(floor(T-289),ceil(P/1e6-1));
mu_Tc2 = mu(ceil(T-289), ceil(P/1e6-1));
mu_Tc  = (mu_Tc2 - mu_Tc1)*(T-floor(T)) + mu_Tc1;

out = (mu_Tc-mu_Tf)*(P/1e6-floor(P/1e6)) + mu_Tf; % (uPa*s) = 10-6 Pa*s
end

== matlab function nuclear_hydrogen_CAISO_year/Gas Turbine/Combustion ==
function T_f = fcn(T_d, m_a, m_f)
eta_comb = 0.99;   % combustor efficiency;
LHV      = 120210; % (kJ/kg) lower heating value of hydrogen https://chemeng.queensu.ca/courses/CHEE332/files/ethanol_heating-values.pdf
C_ph     = 1.157;  % specific heat of hot gas flow (kJ/kg*K)

T_f = T_d + (eta_comb*LHV)/C_ph*m_f/(m_f + m_a);

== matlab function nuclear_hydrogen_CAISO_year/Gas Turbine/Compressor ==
function [Td, m_a, P_out] = fcn(P_amb, theta_IGV, T_amb, m_an)
%% Parameter
gamma_c   = 1.4;    % cold end ratio of specific heats
PR_c      = 15.4;   % pressure ratio
eta_c     = 0.86;   % compressor efficiency
theta_max = 85;     % max IGV angle(degree)
theta_min = 11.6;   % min IGV angle(degree)
P_amb_o   = 1;      % ambient air pressure reference (atm)
T_amb_o   = 288.15; % ambient air temperature reference (K)
%% Function
m_a   = P_amb/P_amb_o*sqrt(T_amb_o/T_amb)*(sind(theta_IGV - theta_min)/sind(theta_max - theta_min))*m_an;
% Air flow rate
x_c   = (PR_c*m_a/m_an)^((gamma_c - 1)/gamma_c);
% 
Td    = T_amb*(1 + (x_c - 1)/eta_c);
% outlet Temp of compressor
P_out = PR_c*P_amb;

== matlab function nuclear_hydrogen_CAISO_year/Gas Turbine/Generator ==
function [P_overall, efficiency] = fcn(m_f, m_a, T_f, T_e, T_d, T_amb)
C_ph = 1.157; % specific heat of hot gas flow (kJ/kg*K)
C_pa = 1.005; % specific heat of air flow (kJ/kg*K)
if m_f<0.05236
    P_overall = 0;
else
    P_overall = ((m_f + m_a)*C_ph*(T_f - T_e) - m_a*C_pa*(T_d - T_amb))*1e-3; % MW
end
if P_overall<0
    P_overall =0;
end
LHV      = 120210; % (kJ/kg) lower heating value of hydrogen https://chemeng.queensu.ca/courses/CHEE332/files/ethanol_heating-values.pdf
efficiency = P_overall*1e3/(m_f*LHV)*100;

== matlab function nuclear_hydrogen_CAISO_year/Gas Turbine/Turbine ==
function T_e = fcn(m_f, T_f, m_a, m_an)
%% Parameters
PR_T    = 15.4; % Expansion ratio
%m_an    = 20;  % nomial exhaust mass flow kg/s
m_fn    = 0.2; % nominal fuel flow (kg/s)
gamma_h = 1.33; % hot end ratio of specific heats
eta_t   = 0.89; % Turbine Efficiency
%% Functions
x_h = (PR_T*(m_f + m_a)/(m_fn + m_an))^((gamma_h - 1)/gamma_h);

T_e = T_f*(1 - (1 - 1/x_h)*eta_t);
% Exhaust gas Temp

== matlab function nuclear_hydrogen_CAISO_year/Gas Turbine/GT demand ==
function GT_demand = fcn(Steam_Turb, grid_demand)
GT_demand = grid_demand - Steam_Turb;
if GT_demand<0
    GT_demand = 0;
end

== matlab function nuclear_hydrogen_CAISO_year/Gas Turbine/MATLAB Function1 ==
function Set_point = fcn(SP, Cavern_Pressure)
if Cavern_Pressure<6.5e6
    Set_point = 0;
else
    Set_point = SP;
end

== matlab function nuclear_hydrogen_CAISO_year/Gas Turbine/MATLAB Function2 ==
function m_H2 = fcn(m_f, GT_SP, Cavern_P)
if GT_SP <0.1
    m_H2 = 0;
% elseif Cavern_P <7e6
%     m_H2 = 0;
else
    m_H2 = m_f;
end

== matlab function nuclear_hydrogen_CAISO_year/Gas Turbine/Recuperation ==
function [Tc_in,T_6] = fcn(T_e, T_d, m_f, m_a)
eff_rec = 0.75;
C_pa = 1.005; % specific heat of air flow (kJ/kg*K)
C_ph = 1.157; % specific heat of hot gas flow (kJ/kg*K)

Tc_in = eff_rec*(T_e-T_d) + T_d;

T_6 = T_e - m_a*C_pa*(Tc_in - T_d)/((m_f+m_a)*C_ph);

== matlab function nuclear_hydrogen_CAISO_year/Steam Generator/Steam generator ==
function [T_steam_out, m_steam]  = fcn(Tmin, mdot_l,Tin0)
coder.extrinsic('XSteam.m');
P_water_in = 127.6;  % inlet pressure of primary side (bar)
P_water_out = 127.6; % outlet pressure of primary side (bar)
H_water_in = XSteam('h_pT', P_water_in, Tmin);   % inlet enthalpy of primary side (kJ/kg)
H_water_out = XSteam('h_pT', P_water_out, Tin0); % outlet enthalpy of primary side (kJ/kg)

T_steam_out = 307.75; % C https://inldigitallibrary.inl.gov/sites/sti/sti/Sort_20117.pdf
H_steam = XSteam('h_pT', 34.6, T_steam_out);
H_water = XSteam('h_pT', 34.6, 38.97);

DelHvap = 2255.18816568; % H_steam - H_water % kJ/kg
m_steam = mdot_l*(H_water_in - H_water_out)/DelHvap;

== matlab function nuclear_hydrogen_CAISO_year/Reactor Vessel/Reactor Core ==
function [dNdt, dCdt, dTfdt, dTmdt, Power, mdot_l] = fcn(N, Tf, Tm, z, C, Tin, beta, ...
    Lambda, alpha_f, Tf0, alpha_m, Tm0, p2, p1, p0, Mf, lambdaC,...
    phi0, m, NA, MW, Ef, sigmaN, As, Mm, h, r_pellet, r_clad)
dNdt = beta*N/Lambda*(alpha_f*(Tf - Tf0) + alpha_m*(Tm - Tm0) ...
    + p2*z^2 + p1*z + p0 + - 1) + C*beta/Lambda; %sigmaX/beta*(X - X0)
dCdt = lambdaC*(N - C);
tau = (Tf + 273.15);
kappa_f = 4.15; % W/(m*C)
kappa_clad = 19.04; % W/(m*C)
U = 1/(1/(h*As)) + r_pellet/(As*kappa_f) + r_clad/(As*kappa_clad) ;
Cpf = 302.27*(548.68/tau)^2*exp(548.68/tau)/(exp(548.68/tau)-1)^2+2*8.463e-3*tau+...
    8.741e-7*18531.7*exp(-18531.7/tau)/tau^2; % (J/kg/K) thermodynamics properties of UO2
Cpm = (-203.6060 + 1523.290*(Tm+273.15)/1000 - 3196.413*((Tm+273.15)/1000)^2 +...
    2474.455*((Tm+273.15)/1000)^3 + 3.855326/((Tm+273.15)/1000)^2)*1000/18.01; % (J/kg/K) NIST thermodynamics properties https://webbook.nist.gov/cgi/cbook.cgi?ID=C7732185&Type=JANAFL&Plot=on
A1 = U/(Mf*Cpf); 
A3 = U/(Mm*Cpm);
mdot_l = 561.7; % kg/s Konor
Power = N/100*phi0*m*NA/MW*Ef*sigmaN*1e-6; % MWt
dTfdt = Power*1e6/(Mf*Cpf) - A1*(Tf - Tm);% + A1*(Tf0 - Tm0)/N0*N; %;
dTmdt = A3*(Tf - Tm) - mdot_l/Mm*(Tm - Tin);%- A3*(Tf0 - Tm0)*(Tm - Tin)/(Tm0 - Tin0);
